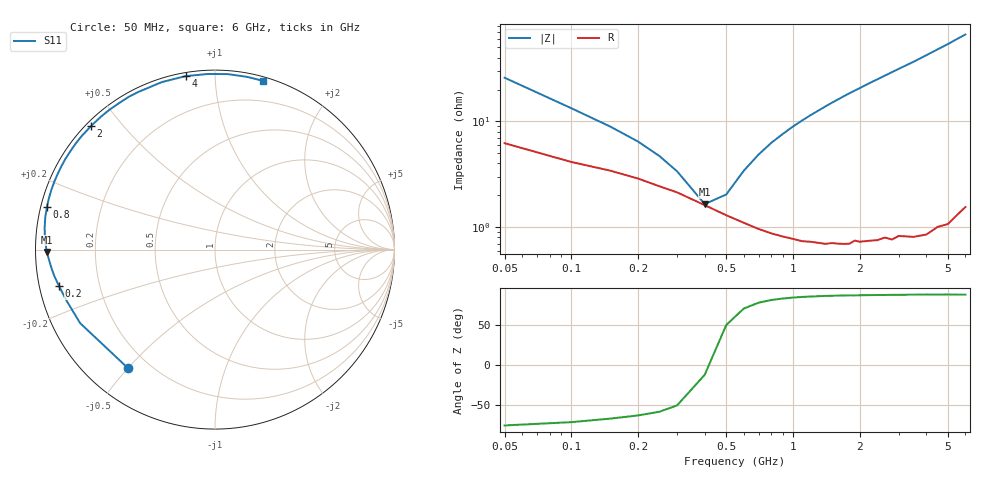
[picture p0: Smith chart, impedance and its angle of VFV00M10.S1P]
! Infineon Technologies  Discrete & RF Semiconductors
! BBY 58-03
! Si Tuning Diode in SOD323
! VR =
! S-Parameters:  June  1999
# GHz  S  MA  R  50
!  f  S11
! GHz  MAG  ANG
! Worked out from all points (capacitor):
!   34 points, 50 MHz to 6 GHz, reference 50 ohm
!   read as one part to ground: C = 118 pF near 50 MHz
!   lowest |Z| = 1.65 ohm at 400 MHz (marker M1)
!   series resonance near 418.2 MHz, so ESL is about 1.2 nH
!   S11 on the Smith chart (normalised r, x): 50 MHz: 0.12, -0.50; 200 MHz: 0.06, -0.12; 800 MHz: 0.02, +0.12; 2 GHz: 0.01, +0.41; 4 GHz: 0.02, +0.84; 6 GHz: 0.03, +1.33
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0.05  0.8197 -126.1
0.1  0.8559 -151.4
0.15  0.8752 -161.2
0.2  0.8924 -166.8
0.25  0.9078 -170.8
0.3  0.9184 -174.0
0.4  0.9375 -179.2
0.5  0.9495 176.4
0.6  0.9571 172.6
0.7  0.9627 169.1
0.8  0.9662 165.8
1  0.9704 159.8
1.2  0.9727 154.3
1.4  0.9745 149.1
1.6  0.975 144.2
1.8  0.9758 139.5
2  0.9754 135.2
2.2  0.9757 130.9
2.4  0.9762 127.0
2.6  0.9756 123.1
2.8  0.9775 119.4
3  0.9766 115.8
3.5  0.9791 107.6
4  0.9803 99.6
4.5  0.9793 92.3
5  0.9804 85.8
5.5  0.9789 79.5
6  0.9778 74.0
